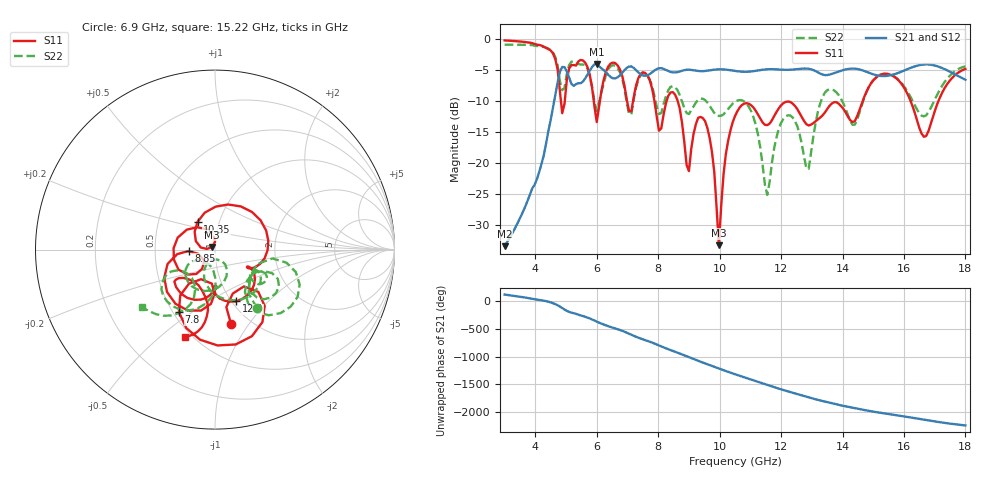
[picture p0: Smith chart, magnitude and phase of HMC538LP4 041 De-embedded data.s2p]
! Chelmsford, MA 01824
! http://www.hittite.com
! Tel: 978-250-3343
! Fax: 978-250-3373
! Device  :  HMC538LP4
! Description:  600 Analog Phase Shifter
! Frequency  :  6.0 GHz - 15.0 GHz
! Package  :  LP4  - 4x4 mm Quad Flatpack No-Lead (QFN) Plastic Package: 24 pin
! Ports  :  2 RF, 1 DC
!  Pin  3  = Rfin  = Port 1
!  Pin  16  = Rfout = Port 2
!  pin  21  = vCTL
! Voltages:  VCTL  = 0 to 5.0 Volts
! Currents :  Vb(V)  Vd(V)  Ib(mA)  Id(mA)
!  0.00  4.10  0.000000	0.480488
! Data:  The device was measured on evaluation board 111296-1.
!  Data was collected using a calibrated network analyzer.
!  The evaluation circuit board was modeled and simulated.This was use
!  to removed the evaluation board circuit from the measured data.
!  The reference plane is the center of the package pin.
! Misc:  Lot #
!Date Measured:  03 - 11 -2009
! Date:  03 - 17 -2009
! Note:
!  Hittite Microwave supplies this data as a sample of measured data at the
!  package pin for this package product.  Your particular data for this product
!  may vary.
!  Data was taken at 25 degrees C.
!  Hittite Microwave reserves the right to change this data at anytime.
# MHz S MA R 50
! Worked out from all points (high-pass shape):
!   201 points, 3 GHz to 18 GHz, reference 50 ohm
!   highest |S21| = -4.01 dB at 6 GHz (marker M1); lowest = -33.4 dB at 3 GHz (marker M2)
!   |S21| within 3 dB of the highest: 4.725 GHz to 5.16 GHz (435.3 MHz wide, 8.81 % of centre); 5.503 GHz to end of sweep
!   lowest |S11| = -33.3 dB at 9.975 GHz (marker M3), VSWR 1.04, Z = 48.4 + j1.42 ohm
!   |S11| at or under -10 dB: 7.878 GHz to 8.273 GHz (395.4 MHz wide, 4.9 % of centre); 8.635 GHz to 14.66 GHz (6.022 GHz wide, 51.7 % of centre); 16.22 GHz to 17.12 GHz (905.1 MHz wide, 5.43 % of centre)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
!   |S22| runs from -25.1 to -0.9 dB; largest |S21 - S12| = 0.0027
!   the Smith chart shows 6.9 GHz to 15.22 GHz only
!   S11 on the Smith chart (normalised r, x): 6.9 GHz: 0.82, -0.83; 7.8 GHz: 0.54, -0.44; 8.85 GHz: 0.74, -0.01; 10.35 GHz: 0.79, +0.25; 12.3 GHz: 1.05, -0.67; 15.22 GHz: 0.46, -0.61
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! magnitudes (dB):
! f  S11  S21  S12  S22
! 3 GHz  -0.2  -33.4  -33.4  -0.9
! 4.8 GHz  -8.4  -5.2  -5.3  -6.8
! 5.55 GHz  -3.4  -6.8  -6.9  -4.1
! 6 GHz  -13.4  -4.0  -4.0  -11.6
! 6.375 GHz  -4.4  -5.7  -5.8  -4.8
! 6.9 GHz  -7.5  -5.0  -5.0  -7.9
! 7.8 GHz  -7.9  -5.4  -5.4  -7.6
! 8.025 GHz  -14.8  -4.7  -4.7  -12.1
! 8.475 GHz  -8.6  -5.4  -5.4  -7.6
! 8.85 GHz  -16.6  -5.0  -5.0  -11.1
! 9.6 GHz  -14.3  -5.1  -5.1  -10.2
! 9.975 GHz  -33.3  -4.9  -4.9  -12.4
! 10.35 GHz  -14.8  -5.0  -5.0  -10.8
! 10.5 GHz  -12.4  -5.1  -5.1  -10.1
! 11.55 GHz  -13.9  -4.8  -4.9  -25.1
! 12.3 GHz  -10.1  -4.9  -4.9  -12.3
! 12.82 GHz  -13.7  -4.7  -4.7  -20.9
! 13.05 GHz  -13.6  -5.0  -5.0  -15.7
! 15.22 GHz  -5.8  -5.9  -5.9  -5.7
! 15.53 GHz  -5.7  -5.9  -5.9  -5.7
! 16.65 GHz  -15.8  -4.1  -4.1  -12.5
! 18 GHz  -4.8  -6.6  -6.6  -4.4
